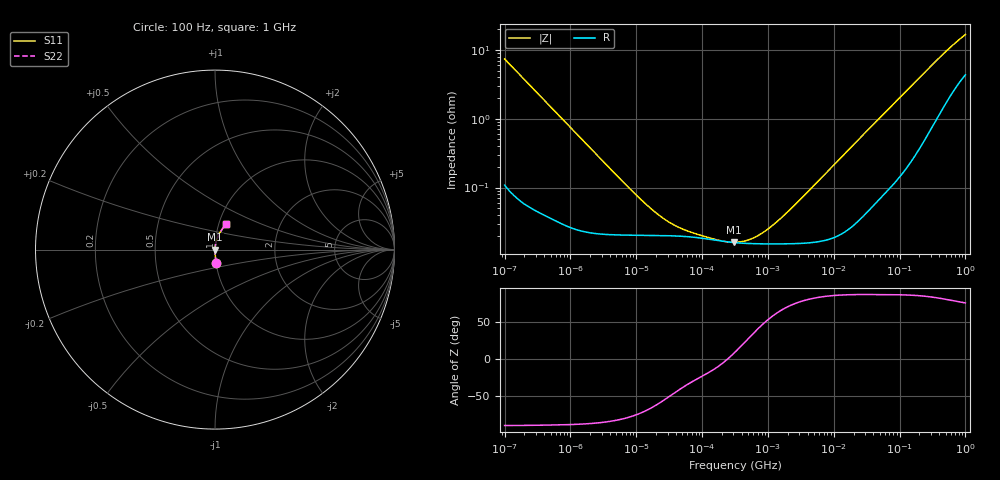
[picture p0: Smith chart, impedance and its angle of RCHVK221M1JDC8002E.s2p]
! RCHVK221M1JDC8002E  S-PARAMETER MODEL  (AEC-Q200 qualified)
! Model Generated by ELNA Corporation (http://www.ty-top.com)
! Version 1.0
! ELNA Control No.240321
! Copyright (c) 2024 ELNA CO.,LTD. All Rights Reserved.
! Products Name : CONDUCTIVE POLYMER HYBRID ALUMINUM ELECTROLYTIC CAPACITORS
! Characteristics :
!  Capacitance  :  220uF  ,  Rated voltage  :  6.3V
!  Operating Temp. Range  :  -55 to +125 degC  ,  Endurance  :  4000hr at 125 degC
!  Dimension D  :  6.3mm  ,  Dimension L  :  5.8mm
! Frequency Range : 100Hz - 1GHz
! External Node Assignments :
!  1  o---| |---o  2
# MHz S RI R 50
!Freq[MHz].  S11 Real  S11 Imag  S21 Real  S21 Imag  S12 Real  S12 Imag  S22 Real  S22 Imag
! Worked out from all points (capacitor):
!   401 points, 100 Hz to 1 GHz, reference 50 ohm
!   read as one part in series: C = 216 uF near 108 Hz
!   lowest |Z| = 16 mohm at 303.7 kHz (marker M1)
!   series resonance near 245.5 kHz, so ESL is about 1.9 nH
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0.0001  0.00648 -0.0732  0.9935 0.0732  0.9935 0.0732  0.00648 -0.0732
0.000113  0.00518 -0.065  0.9948 0.065  0.9948 0.065  0.00518 -0.065
0.000309  0.00102 -0.0239  0.999 0.0239  0.999 0.0239  0.00102 -0.0239
0.001488  0.000258 -0.00503  0.9997 0.00503  0.9997 0.00503  0.000258 -0.00503
0.00912  0.000204 -0.000823  0.9998 0.000823  0.9998 0.000823  0.000204 -0.000823
0.014791  0.000202 -0.000509  0.9998 0.000509  0.9998 0.000509  0.000202 -0.000509
0.022131  0.000201 -0.000342  0.9998 0.000342  0.9998 0.000342  0.000201 -0.000342
0.035892  0.000199 -0.000214  0.9998 0.000214  0.9998 0.000214  0.000199 -0.000214
0.060604  0.000193 -0.00013  0.9998 0.00013  0.9998 0.00013  0.000193 -0.00013
0.165959  0.000171 -3.51e-05  0.9998 3.51e-05  0.9998 3.51e-05  0.000171 -3.51e-05
0.303739  0.000159 2.09e-05  0.9998 -2.09e-05  0.9998 -2.09e-05  0.000159 2.09e-05
0.316228  0.000158 2.5e-05  0.9998 -2.5e-05  0.9998 -2.5e-05  0.000158 2.5e-05
0.533949  0.000154 8.73e-05  0.9998 -8.73e-05  0.9998 -8.73e-05  0.000154 8.73e-05
0.707946  0.000153 0.00013  0.9998 -0.00013  0.9998 -0.00013  0.000153 0.00013
0.938642  0.000152 0.000184  0.9998 -0.000184  0.9998 -0.000184  0.000152 0.000184
1.788546  0.000152 0.000372  0.9998 -0.000372  0.9998 -0.000372  0.000152 0.000372
4.704354  0.00016 0.000995  0.9998 -0.000995  0.9998 -0.000995  0.00016 0.000995
69.9842  0.00116 0.0141  0.9988 -0.0141  0.9988 -0.0141  0.00116 0.0141
184.0772  0.00451 0.036  0.9955 -0.036  0.9955 -0.036  0.00451 0.036
412.0975  0.0177 0.0755  0.9823 -0.0755  0.9823 -0.0755  0.0177 0.0755
695.825  0.0401 0.1141  0.9599 -0.1141  0.9599 -0.1141  0.0401 0.1141
1000  0.0639 0.1449  0.9361 -0.1449  0.9361 -0.1449  0.0639 0.1449
